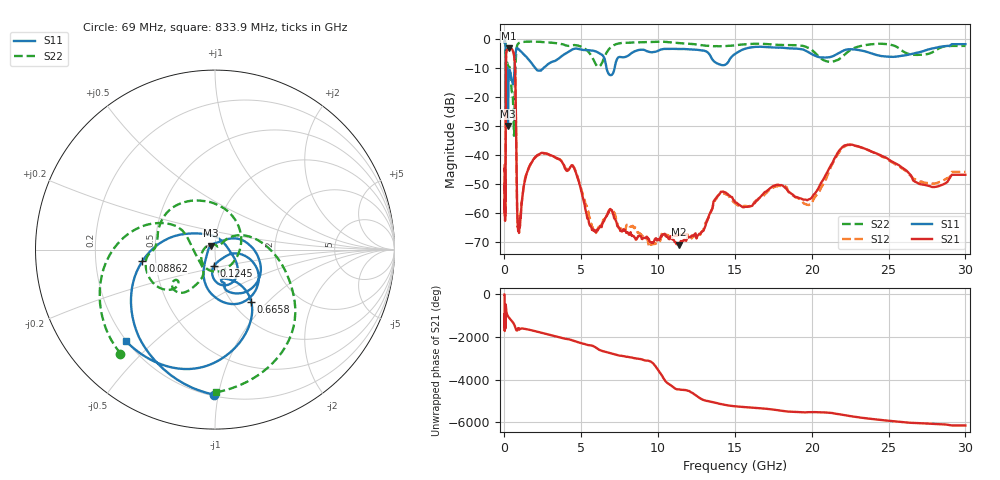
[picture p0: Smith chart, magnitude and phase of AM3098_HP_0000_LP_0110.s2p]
! Date/Time: Thu, Feb 28, 2019 8:30 AM
! Network Analyzer: Agilent Technologies E8364B Rev: A.07.50.67
! Sweep from 0.010 to 30.000 GHz, 1601 Points, Sweep Type: LOG
! Power Supply: 5.022 V, 0.002 A
# Hz S DB R 50
!freq MagS11 AngS11 MagS21 AngS21 MagS12 AngS12 MagS22 AngS22
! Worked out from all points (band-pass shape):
!   1601 points, 10 MHz to 30 GHz, reference 50 ohm
!   highest |S21| = -3.08 dB at 266.5 MHz (marker M1); lowest = -71.0 dB at 11.36 GHz (marker M2)
!   |S21| within 3 dB of the highest: 103.6 MHz to 640.3 MHz (536.8 MHz wide, 144 % of centre)
!   lowest |S11| = -29.9 dB at 225.9 MHz (marker M3), VSWR 1.07, Z = 47.7 + j2.1 ohm
!   |S11| at or under -10 dB: 176.1 MHz to 655.5 MHz (479.4 MHz wide, 115 % of centre); 2.029 GHz to 2.52 GHz (491.3 MHz wide, 21.6 % of centre); 6.648 GHz to 7.164 GHz (516.4 MHz wide, 7.48 % of centre)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
!   |S22| runs from -33.3 to -0.5 dB; largest |S21 - S12| = 0.013
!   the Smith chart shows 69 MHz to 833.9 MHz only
!   S11 on the Smith chart (normalised r, x): 69 MHz: 0.21, -0.97; 88.62 MHz: 0.42, -0.06; 124.5 MHz: 0.97, -0.17; 665.8 MHz: 1.21, -0.81; 833.9 MHz: 0.20, -0.41
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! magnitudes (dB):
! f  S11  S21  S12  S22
! 10 MHz  -0.3  -45.2  -43.0  -0.5
! 38.04 MHz  -0.5  -60.1  -57.8  -0.9
! 69 MHz  -1.9  -50.8  -51.3  -2.1
! 88.62 MHz  -7.8  -19.0  -19.0  -9.1
! 97.94 MHz  -24.0  -7.8  -7.8  -17.5
! 124.5 MHz  -21.0  -4.2  -4.2  -10.8
! 144.7 MHz  -13.0  -3.6  -3.6  -10.1
! 185.8 MHz  -11.3  -3.5  -3.5  -8.1
! 225.9 MHz  -29.9  -3.2  -3.1  -9.5
! 266.5 MHz  -14.4  -3.1  -3.1  -9.7
! 550.5 MHz  -15.5  -3.9  -3.9  -20.4
! 620.7 MHz  -13.1  -5.3  -5.2  -33.2
! 665.8 MHz  -9.0  -7.7  -7.7  -22.2
! 833.9 MHz  -3.0  -59.6  -60.1  -2.0
! 2.084 GHz  -10.4  -40.3  -40.4  -0.8
! 4.458 GHz  -3.3  -43.8  -43.6  -1.9
! 5.812 GHz  -3.9  -65.7  -66.1  -7.2
! 7.926 GHz  -5.9  -66.9  -64.4  -1.1
! 11.36 GHz  -3.3  -71.0  -67.6  -1.2
! 19.8 GHz  -4.4  -55.3  -57.2  -3.0
! 22.56 GHz  -3.4  -36.3  -36.4  -3.5
! 30 GHz  -1.6  -46.8  -45.8  -2.2
